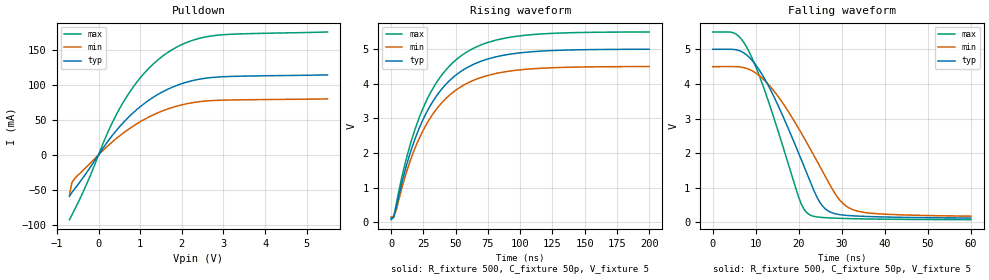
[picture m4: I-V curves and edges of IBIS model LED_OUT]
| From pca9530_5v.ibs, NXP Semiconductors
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[Model]   LED_OUT
Model_type Open_drain
Vref=3.5
Vmeas=1.5
Rref=500
Cref=50p
C_comp   5p   4.8p   5.2p
[Temperature Range] 27   85   -40
[Voltage Range]   5   4.5   5.5
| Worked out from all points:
|   slope of the pulldown table from 0 to 0.75 V, typ, clamps not added: 13.5 ohm
|   falling waveform, R_fixture 500, C_fixture 50p, V_fixture 5: 20-80 % time 10.3ns typ, 12.2ns min, 8.61ns max; typ from 5 V to 0.128 V
|   rising waveform, R_fixture 500, C_fixture 50p, V_fixture 5: 20-80 % time 35.4ns typ, 35.4ns min, 35.3ns max; typ from 0.11 V to 5 V
[Pulldown]
-700mV    -59.59mA   -57.04mA   -92.81mA
-640mV    -53.78mA   -39.6mA    -86.14mA
-570mV    -48.42mA   -33.52mA   -77.9mA
-260mV    -23.08mA   -15.55mA   -38.25mA
240mV     20.6mA     13.69mA    34.51mA
550mV     43.16mA    29.13mA    70.76mA
800mV     58.34mA    39.79mA    94.26mA
1.05V     71.11mA    48.96mA    113.5mA
1.55V     90.43mA    63.09mA    141.6mA
2.12V     104mA      73.05mA    160.7mA
2.74V     110.7mA    77.57mA    170.2mA
5.5V      114.3mA    79.96mA    175.7mA
[Falling Waveform]
R_fixture=500
C_fixture=50p
V_fixture=5
V_fixture_min=4.5
V_fixture_max=5.5
0s        5V         4.5V       5.5V
4.848ns   4.996V     4.501V     5.476V
7.879ns   4.837V     4.448V     5.062V
13.33ns   3.852V     3.931V     3.351V
20ns      1.988V     2.705V     719.9mV
22.42ns   1.25V      2.177V     227.9mV
26.06ns   403.3mV    1.354V     138.8mV
29.09ns   234.1mV    713.7mV    120.7mV
32.12ns   194.5mV    393.5mV    109.7mV
60ns      127.5mV    181.2mV    79.76mV
[Rising Waveform]
R_fixture=500
C_fixture=50p
V_fixture=5
V_fixture_min=4.5
V_fixture_max=5.5
0s        109.9mV    149.5mV    71.11mV
2.02ns    141.6mV    169.1mV    144mV
4.04ns    431.3mV    352.1mV    532mV
14.14ns   1.92V      1.699V     2.153V
24.24ns   2.925V     2.611V     3.249V
38.38ns   3.809V     3.414V     4.209V
54.55ns   4.368V     3.923V     4.816V
72.73ns   4.691V     4.217V     5.166V
98.99ns   4.89V      4.399V     5.381V
200ns     4.998V     4.498V     5.498V
[Ramp]
R_load=500
dV/dt_r   2.934E+0/1.129E-9   2.900E+0/1.498E-9   2.961E+0/8.466E-10
dV/dt_f   2.934E+0/8.416E-9   2.900E+0/1.086E-8   2.961E+0/6.634E-9
|[End   LED_OUT
